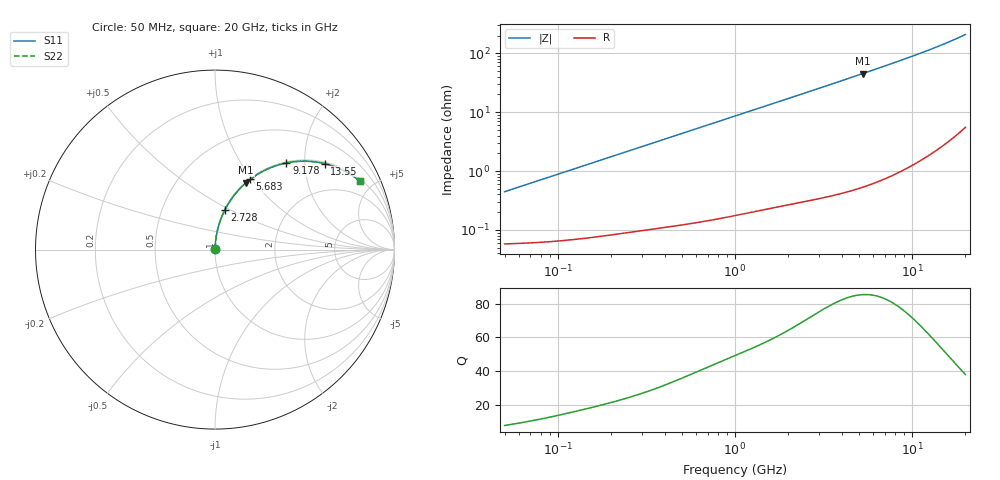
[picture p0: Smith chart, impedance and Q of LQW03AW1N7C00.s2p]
!Murata Part Number: LQW03AW1N7C00
!These Parameters are Measured in Series Mode Connection
!  o--[Z]--o
!Port1  Port2
!  o-------o
!Freq. Start=50[MHz] Stop=20[GHz], 401[Steps]
# Hz S RI R 50
!Freq.(Hz) S11(Real) S11(Imag) S21(Real) S21(Imag) S12(Real) S12(Imag) S22(Real) S22(Imag)
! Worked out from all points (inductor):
!   401 points, 50 MHz to 20 GHz, reference 50 ohm
!   read as one part in series: L = 1.4 nH near 51.52 MHz
!   highest Q = 85.4 at 5.273 GHz (marker M1), where L = 1.37 nH
!   S11 on the Smith chart (normalised r, x): 50 MHz: 1.00, +0.01; 2.728 GHz: 1.01, +0.47; 5.683 GHz: 1.01, +0.98; 9.178 GHz: 1.02, +1.62; 13.55 GHz: 1.04, +2.52; 20 GHz: 1.11, +4.18
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5e7  0.000596 0.00441  0.9994 -0.00441  0.9994 -0.00441  0.000596 0.00441
5.152053e7  0.000599 0.00455  0.9994 -0.00455  0.9994 -0.00455  0.000599 0.00455
1.364002e8  0.000851 0.012  0.9991 -0.012  0.9991 -0.012  0.000851 0.012
3.721004e8  0.0021 0.0321  0.9979 -0.0321  0.9979 -0.0321  0.0021 0.0321
6.380365e8  0.00436 0.0547  0.9956 -0.0547  0.9956 -0.0547  0.00436 0.0547
1e9  0.00902 0.0849  0.991 -0.0849  0.991 -0.0849  0.00902 0.0849
1.689197e9  0.0227 0.1408  0.9773 -0.1408  0.9773 -0.1408  0.0227 0.1408
2.146657e9  0.035 0.1765  0.965 -0.1765  0.965 -0.1765  0.035 0.1765
2.728004e9  0.0542 0.2197  0.9458 -0.2197  0.9458 -0.2197  0.0542 0.2197
3.314454e9  0.0771 0.2605  0.9229 -0.2605  0.9229 -0.2605  0.0771 0.2605
3.908127e9  0.1036 0.2986  0.8964 -0.2986  0.8964 -0.2986  0.1036 0.2986
4.539627e9  0.1346 0.3354  0.8654 -0.3354  0.8654 -0.3354  0.1346 0.3354
5.273168e9  0.1736 0.3729  0.8264 -0.3729  0.8264 -0.3729  0.1736 0.3729
5.683258e9  0.1964 0.3915  0.8036 -0.3915  0.8036 -0.3915  0.1964 0.3915
6.503449e9  0.2434 0.4233  0.7566 -0.4233  0.7566 -0.4233  0.2434 0.4233
7.442007e9  0.2983 0.4514  0.7017 -0.4514  0.7017 -0.4514  0.2983 0.4514
9.178299e9  0.3981 0.4829  0.6019 -0.4829  0.6019 -0.4829  0.3981 0.4829
1.115139e10  0.5026 0.4926  0.4974 -0.4926  0.4974 -0.4926  0.5026 0.4926
1.354865e10  0.6112 0.4789  0.3888 -0.4789  0.3888 -0.4789  0.6112 0.4789
1.621653e10  0.7079 0.4445  0.2921 -0.4445  0.2921 -0.4445  0.7079 0.4445
1.88369e10  0.7811 0.4014  0.2189 -0.4014  0.2189 -0.4014  0.7811 0.4014
2e10  0.8079 0.381  0.1921 -0.381  0.1921 -0.381  0.8079 0.381
